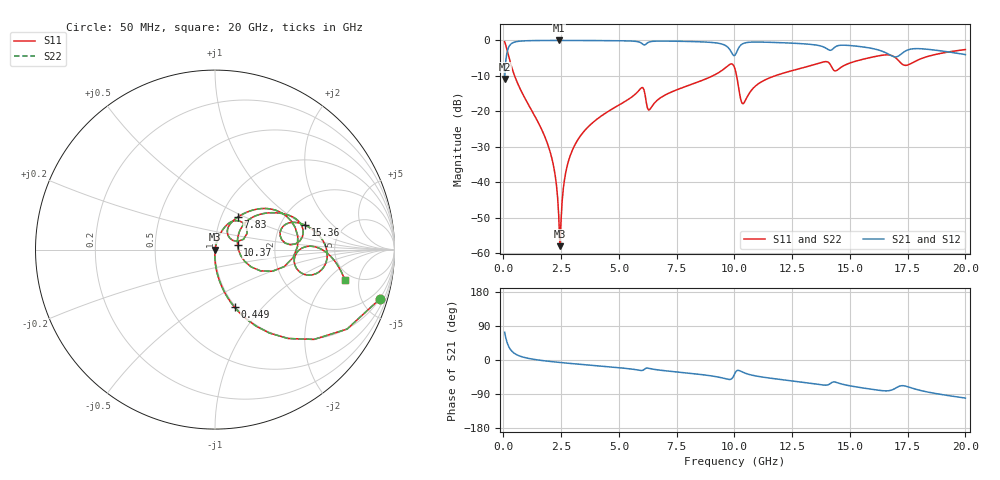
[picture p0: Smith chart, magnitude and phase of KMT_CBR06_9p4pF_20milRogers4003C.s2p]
! Data measured by Modelithics Inc. support@modelithics.com 813-866-6335
! KEMET CBR0603 9.4pF, Pad Width= 0.851mm, Pad Length= 0.64mm, Pad Gap= 0.62mm, 20mil Rogers 4003C substrate Data, January 2022
# hz S ma R 50
! 2 Port Network Data from SP1.SP block
! freq  magS11  angS11  magS21  angS21  magS12  angS12  magS22  angS22
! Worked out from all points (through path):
!   401 points, 50 MHz to 20 GHz, reference 50 ohm
!   highest |S21| = -0.01 dB at 2.394 GHz (marker M1); lowest = -10.9 dB at 50 MHz (marker M2)
!   group delay of S21, straight-line fit = 14.5 ps
!   lowest |S11| = -58.0 dB at 2.444 GHz (marker M3), VSWR 1.00, Z = 50.1 - j0.0351 ohm
!   |S11| at or under -10 dB: 484.6 MHz to 9.053 GHz (8.568 GHz wide, 180 % of centre); 10.09 GHz to 11.75 GHz (1.652 GHz wide, 15.1 % of centre)
!   |S22| runs from -58.0 to -0.4 dB; largest |S21 - S12| = 0
!   S11 on the Smith chart (normalised r, x): 50 MHz: 0.99, -6.66; 449 MHz: 0.99, -0.72; 7.83 GHz: 1.20, +0.46; 10.37 GHz: 1.29, +0.06; 15.36 GHz: 2.75, +1.02; 20 GHz: 4.22, -3.25
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5e7  0.9583 -16.7  0.2854 73.3  0.2854 73.3  0.9583 -16.7
2.495e8  0.5542 -56.9  0.8317 33.0  0.8317 33.0  0.5542 -56.9
4.49e8  0.34 -71.2  0.9397 18.7  0.9397 18.7  0.34 -71.2
1.94525e9  0.03229 -91.3  0.9983 -3.3  0.9983 -3.3  0.03229 -91.3
2.194625e9  0.01534 -90.5  0.9986 -5.0  0.9986 -5.0  0.01534 -90.5
2.394125e9  0.003343 -74.6  0.9987 -6.2  0.9987 -6.2  0.003343 -74.6
2.444e9  0.001263 -16.1  0.9987 -6.5  0.9987 -6.5  0.001263 -16.1
2.793125e9  0.01882 77.4  0.9984 -8.5  0.9984 -8.5  0.01882 77.4
3.391625e9  0.04792 76.4  0.9973 -11.8  0.9973 -11.8  0.04792 76.4
5.93525e9  0.2093 49.5  0.932 -27.6  0.932 -27.6  0.2093 49.5
6.33425e9  0.1064 45.8  0.9556 -22.5  0.9556 -22.5  0.1064 45.8
6.73325e9  0.1502 59.6  0.9784 -26.5  0.9784 -26.5  0.1502 59.6
7.8305e9  0.221 55.0  0.9695 -33.5  0.9695 -33.5  0.221 55.0
9.576125e9  0.4029 33.0  0.8594 -48.9  0.8594 -48.9  0.4029 33.0
1.0025e10  0.397 -13.8  0.6186 -34.6  0.6186 -34.6  0.397 -13.8
1.037412e10  0.1281 10.7  0.9023 -32.5  0.9023 -32.5  0.1281 10.7
1.127188e10  0.2723 40.9  0.9453 -45.6  0.9453 -45.6  0.2723 40.9
1.336662e10  0.4474 25.7  0.8747 -61.8  0.8747 -61.8  0.4474 25.7
1.536162e10  0.5218 15.0  0.8247 -71.9  0.8247 -71.9  0.5218 15.0
1.670825e10  0.6231 -6.5  0.6311 -80.8  0.6311 -80.8  0.6231 -6.5
1.74065e10  0.445 -7.0  0.7092 -68.9  0.7092 -68.9  0.445 -7.0
2e10  0.7441 -13.4  0.6312 -100.5  0.6312 -100.5  0.7441 -13.4
